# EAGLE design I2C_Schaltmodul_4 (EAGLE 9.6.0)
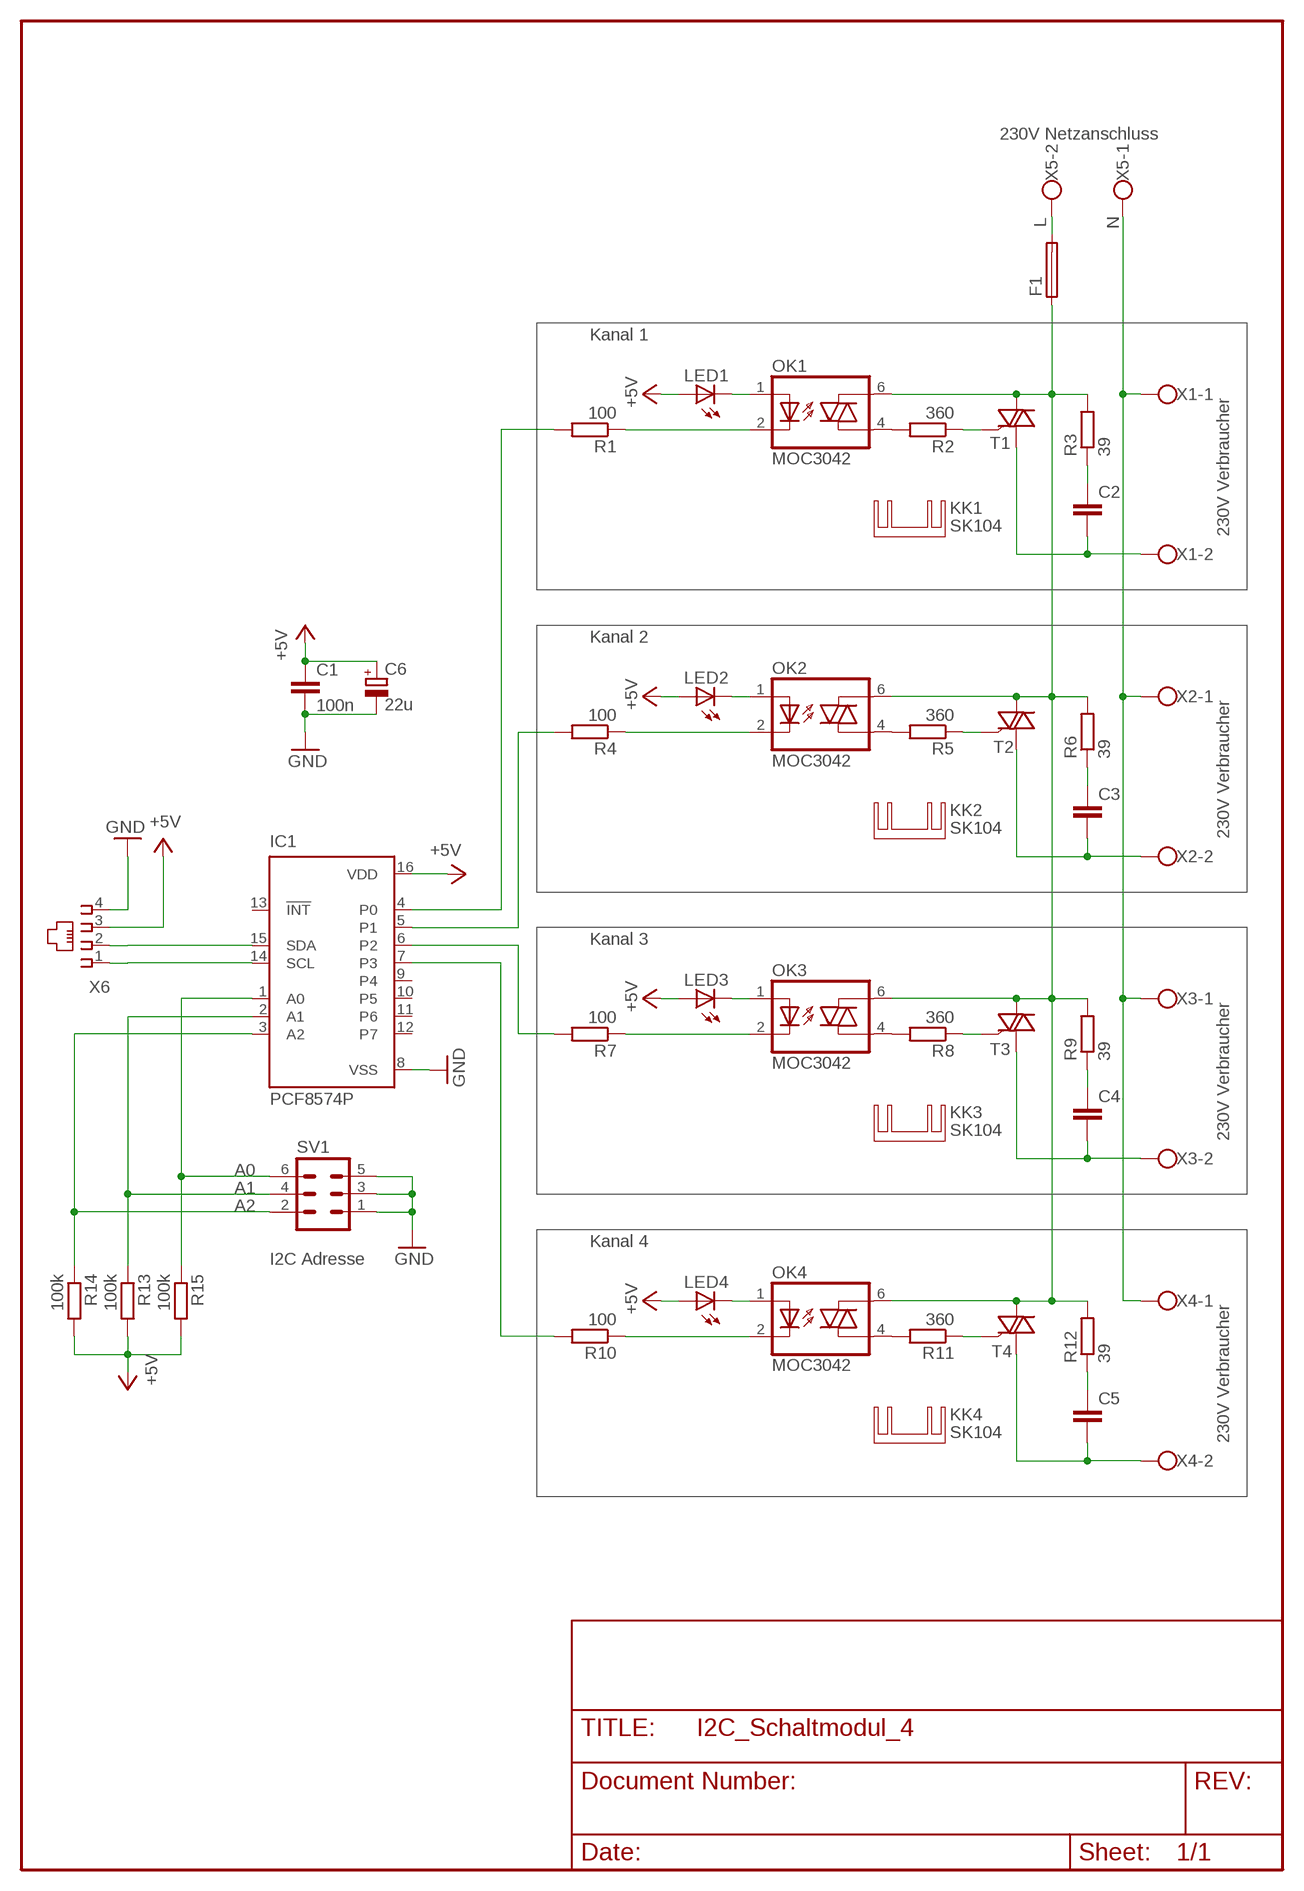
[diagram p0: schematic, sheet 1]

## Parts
C1  100n  C-EU075-032X103  [C075-032X103]
C2  C-EU102-043X133  [C102-043X133]
C3  C-EU102-043X133  [C102-043X133]
C4  C-EU102-043X133  [C102-043X133]
C5  C-EU102-043X133  [C102-043X133]
C6  22u  CPOL-EUE2.5-5  [E2,5-5]
F1  SH25  [SH25]
IC1  PCF8574P  [DIL16]
KK1  SK104  [SK104]
KK2  SK104  [SK104]
KK3  SK104  [SK104]
KK4  SK104  [SK104]
LED1  LED3MM  [LED3MM]
LED2  LED3MM  [LED3MM]
LED3  LED3MM  [LED3MM]
LED4  LED3MM  [LED3MM]
OK1  MOC3042  IL420  [DIL06]
OK2  MOC3042  IL420  [DIL06]
OK3  MOC3042  IL420  [DIL06]
OK4  MOC3042  IL420  [DIL06]
R1  100  R-EU_0207/10  [0207/10]
R2  360  R-EU_0207/10  [0207/10]
R3  39  R-EU_0411/15  [0411/15]
R4  100  R-EU_0207/10  [0207/10]
R5  360  R-EU_0207/10  [0207/10]
R6  39  R-EU_0411/15  [0411/15]
R7  100  R-EU_0207/10  [0207/10]
R8  360  R-EU_0207/10  [0207/10]
R9  39  R-EU_0411/15  [0411/15]
R10  100  R-EU_0207/10  [0207/10]
R11  360  R-EU_0207/10  [0207/10]
R12  39  R-EU_0411/15  [0411/15]
R13  100k  R-EU_0207/10  [0207/10]
R14  100k  R-EU_0207/10  [0207/10]
R15  100k  R-EU_0207/10  [0207/10]
SV1  MA03-2  [MA03-2]
T1  TIC225SBVH  [TO220BVH]
T2  TIC225SBVH  [TO220BVH]
T3  TIC225SBVH  [TO220BVH]
T4  TIC225SBVH  [TO220BVH]
X1  W237-102  [W237-102]
X2  W237-102  [W237-102]
X3  W237-102  [W237-102]
X4  W237-102  [W237-102]
X5  W237-102  [W237-102]
X6  215876-6  [215876-6]

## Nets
+5V: C1.1 C6.+ IC1.16(VDD) LED1.A LED2.A LED3.A LED4.A R13.2 R14.2 R15.2 X6.3
A0: IC1.1(A0) R15.1 SV1.6
A1: IC1.2(A1) R13.1 SV1.4
A2: IC1.3(A2) R14.1 SV1.2
GND: C1.2 C6.- IC1.8(VSS) SV1.1 SV1.3 SV1.5 X6.4
L: F1.2 X5.2
N: X1.1 X2.1 X3.1 X4.1 X5.1
N$1: IC1.4(P0) R1.2
N$2: LED1.K(C) OK1.1(A)
N$3: OK1.4(A1) R2.2
N$4: IC1.5(P1) R4.2
N$5: R2.1 T1.3(G)
N$6: C2.1 R3.1
N$7: OK1.2(C) R1.1
N$8: OK2.4(A1) R5.2
N$9: OK3.4(A1) R8.2
N$10: OK4.4(A1) R11.2
N$11: C3.2 T2.1(A1) X2.2
N$12: C3.1 R6.1
N$13: C2.2 T1.1(A1) X1.2
N$14: LED2.K(C) OK2.1(A)
N$15: OK2.2(C) R4.1
N$16: R5.1 T2.3(G)
N$17: C4.2 T3.1(A1) X3.2
N$18: C4.1 R9.1
N$19: IC1.6(P2) R7.2
N$20: LED3.K(C) OK3.1(A)
N$21: OK3.2(C) R7.1
N$22: R11.1 T4.3(G)
N$24: C5.2 T4.1(A1) X4.2
N$25: C5.1 R12.1
N$26: IC1.7(P3) R10.2
N$27: LED4.K(C) OK4.1(A)
N$28: OK4.2(C) R10.1
N$29: R8.1 T3.3(G)
N$100: F1.1 OK1.6(A2) OK2.6(A2) OK3.6(A2) OK4.6(A2) R3.2 R6.2 R9.2 R12.2 T1.2(A2) T2.2(A2) T3.2(A2) T4.2(A2)
SCL: IC1.14(SCL) X6.2
SDA: IC1.15(SDA) X6.1
Unconnected: IC1.9(P4) IC1.10(P5) IC1.11(P6) IC1.12(P7) IC1.13(!INT)

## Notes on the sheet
- 230V Netzanschluss
- Kanal 1
- 230V Verbraucher
- Kanal 2
- 230V Verbraucher
- Kanal 3
- 230V Verbraucher
- Kanal 4
- I2C Adresse
- 230V Verbraucher

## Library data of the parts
C1-C5 = rcl:C-EU: CAPACITOR, European symbol
C6 = rcl:CPOL-EU: POLARIZED CAPACITOR, European symbol
F1 = fuse:SH25: FUSE HOLDER
IC1 = micro-philips:PCF8574: I2C-Bus I/O DEVICE
KK1-KK4 = heatsink:SK104: HEATSINK
LED1-LED4 = led:LED: LED
OK1-OK4 = optocoupler:IL420: SIEMENS OPTO COUPLER
R1-R15 = rcl:R-EU_: RESISTOR, European symbol
SV1 = con-lstb:MA03-2: PIN HEADER
T1-T4 = selfmade:TIC225S: TRIAC
X1-X5 = con-wago-500:W237-102: WAGO SCREW CLAMP
X6 = con-amp:215876-6: AMP connector

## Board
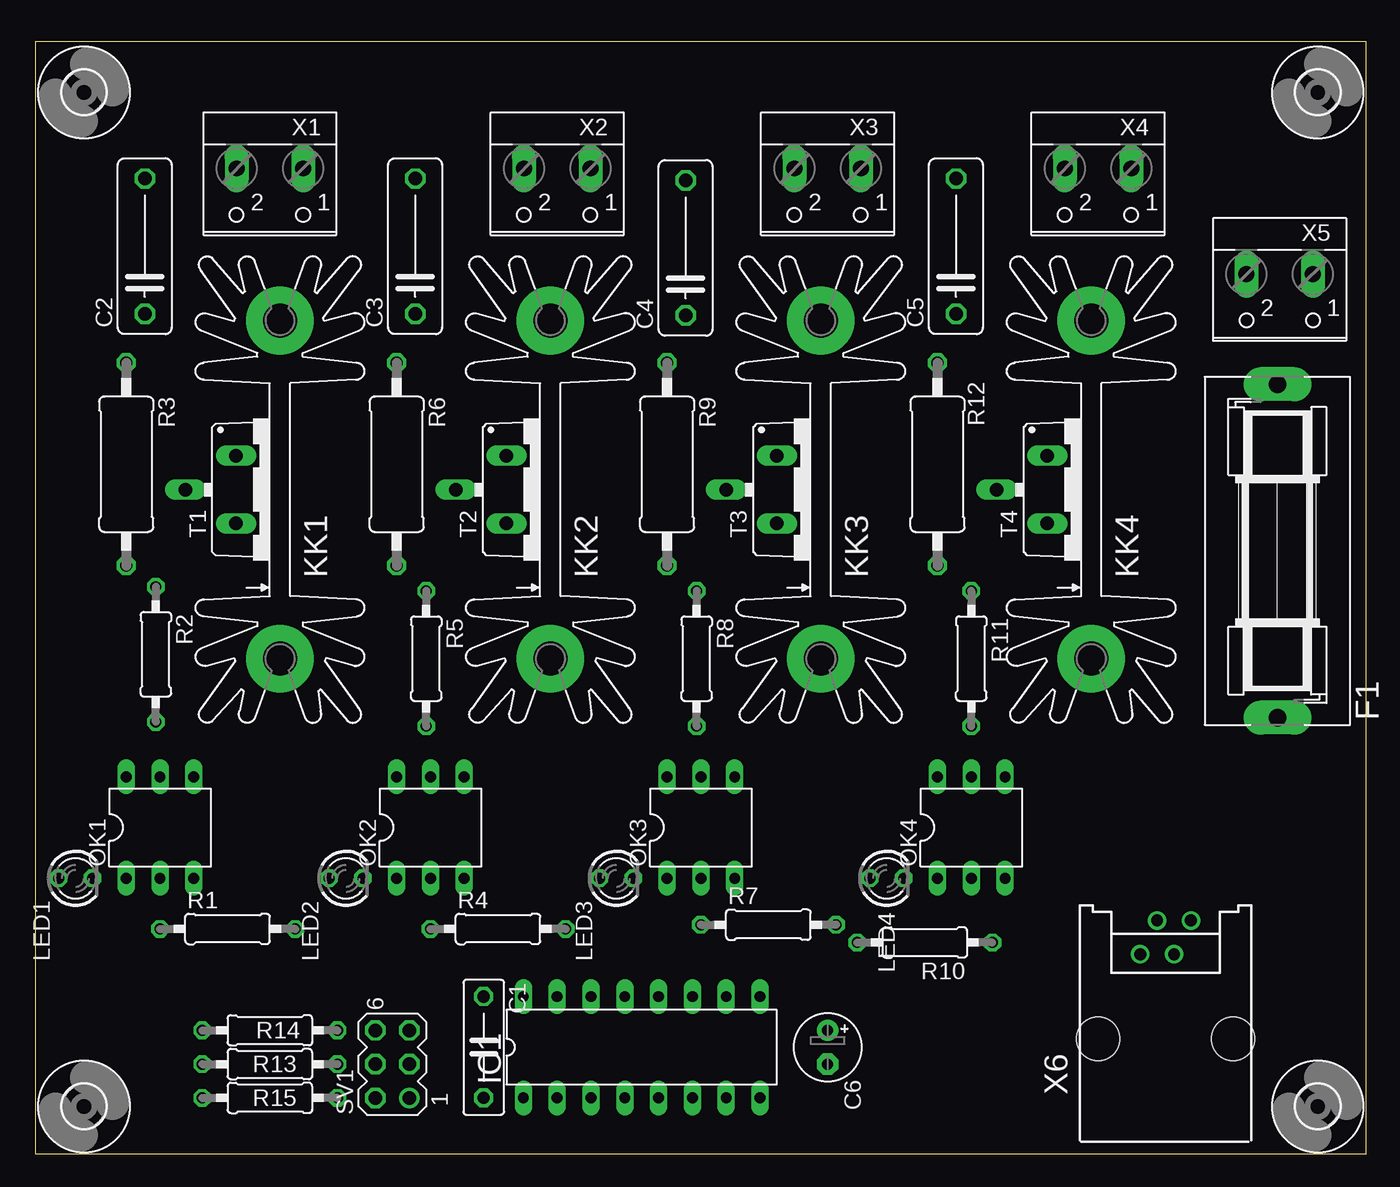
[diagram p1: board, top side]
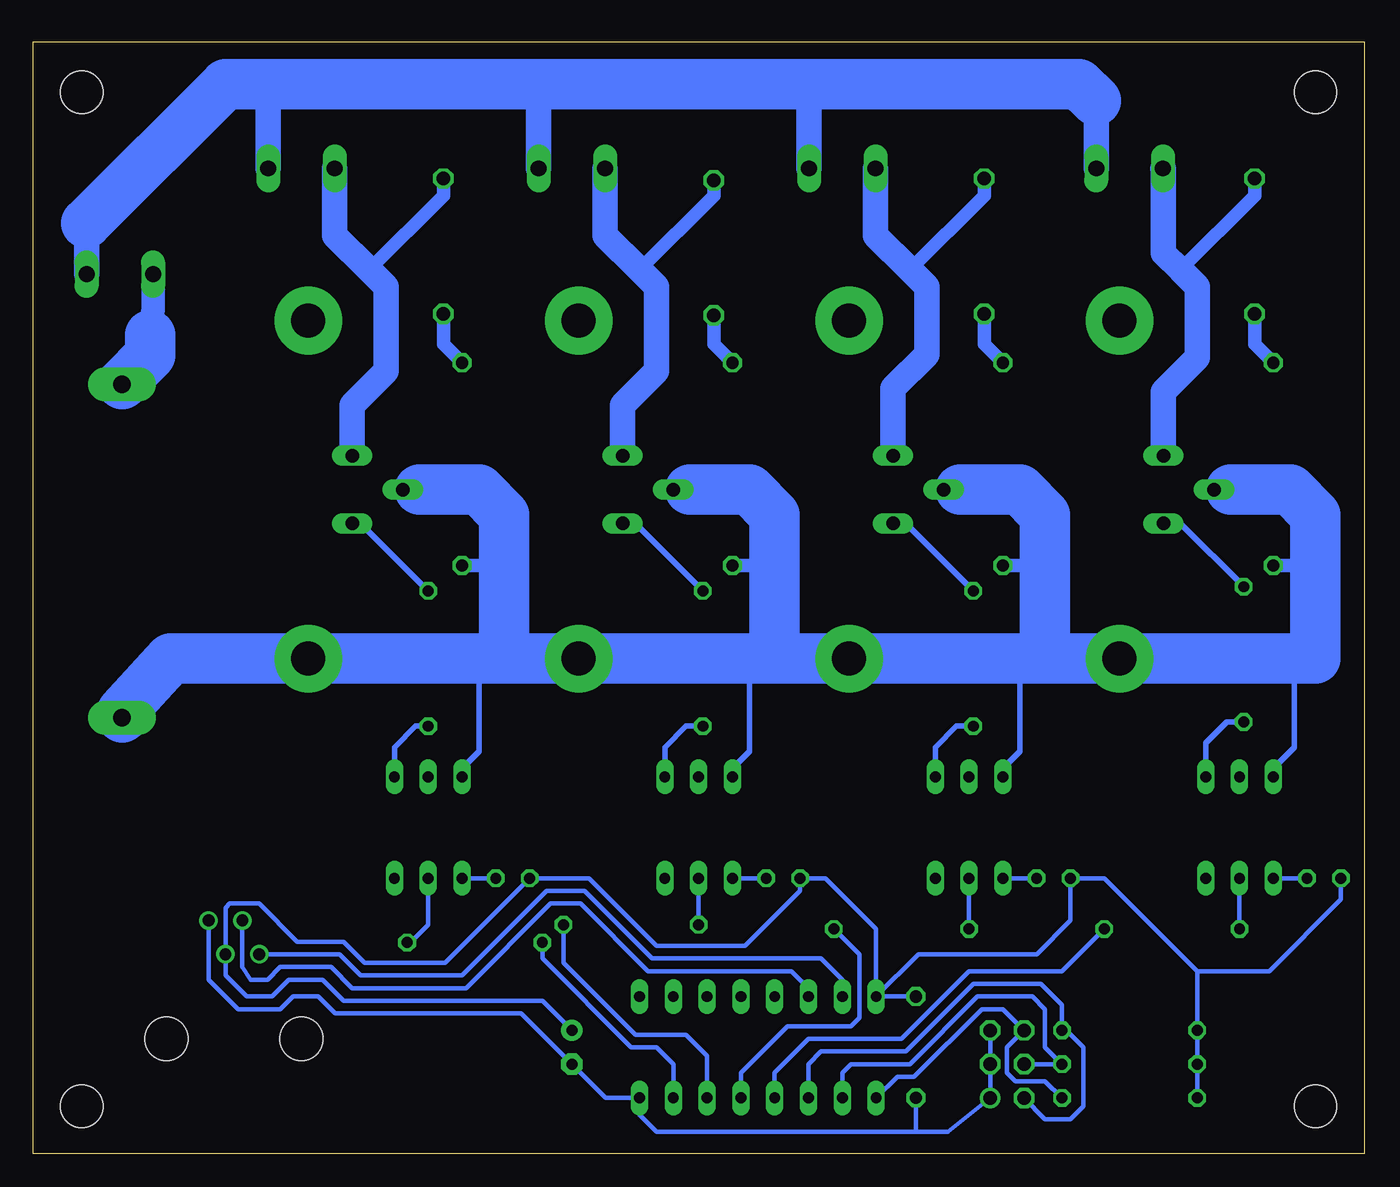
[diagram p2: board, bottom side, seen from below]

Size 100 x 83.56 mm. Coordinates in mm from the lower left corner, seen from the top.
Outline: 0,0 100,0 100,83.56 0,83.56 0,0
Copper layers (1*16): Top 0.035mm / dielectric 1.5mm / Bottom 0.035mm
Design rules "default": minimum track width 12mil, minimum drill 24mil, track to track 12mil, track to pad 12mil, pad to pad 12mil, via to via 12mil, smd to smd 8mil, copper to edge 40mil, drill to drill 8mil, minimum pad ring 10mil, minimum via ring 8mil, stop-mask expansion 4mil, vias tented up to drill 0mil, thermal gap 10mil

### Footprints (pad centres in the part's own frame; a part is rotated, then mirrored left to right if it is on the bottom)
C075-032X103 = drill 0.914 octagon: 1 -3.81,0; 2 3.81,0
C102-043X133 = drill 1.016 octagon: 1 -5.08,0; 2 5.08,0
E2,5-5 = drill 0.813 pad 1.6: + -1.27,0 | drill 0.813 pad 1.6 octagon: - 1.27,0
SH25 = drill 1.321 pad 2.54 long: 1 -12.522,0; 2 12.522,0
DIL16 = drill 0.813 long: 1 -8.89,-3.81; 2 -6.35,-3.81; 3 -3.81,-3.81; 4 -1.27,-3.81; 5 1.27,-3.81; 6 3.81,-3.81; 7 6.35,-3.81; 8 8.89,-3.81; 9 8.89,3.81; 10 6.35,3.81; 11 3.81,3.81; 12 1.27,3.81; 13 -1.27,3.81; 14 -3.81,3.81; 15 -6.35,3.81; 16 -8.89,3.81
SK104 = drill 2.54 pad 5.08: A2,5 -12.7,-0.762; B2,5 12.7,-0.762
LED3MM = drill 0.813 octagon: A -1.27,0; K 1.27,0
DIL06 = drill 0.813 long: 1 -2.54,-3.81; 2 0,-3.81; 3 2.54,-3.81; 4 2.54,3.81; 5 0,3.81; 6 -2.54,3.81
0207/10 = drill 0.813 octagon: 1 -5.08,0; 2 5.08,0
0411/15 = drill 0.914 octagon: 1 -7.62,0; 2 7.62,0
MA03-2 = drill 1.016: 1 -2.54,-1.27 | drill 1.016 octagon: 2 -2.54,1.27; 3 0,-1.27; 4 0,1.27; 5 2.54,-1.27; 6 2.54,1.27
TO220BVH = drill 1.016 long: 1 -2.54,-2.54; 2 0,-6.35; 3 2.54,-2.54
3,2 = hole 3.2: 0,0
W237-102 = drill 1.194 long: 1 -2.5,-1.27; 2 2.5,-1.27
215876-6 = drill 0.889: 1 -1.905,6.35; 2 -0.635,8.89; 3 0.635,6.35; 4 1.905,8.89 | hole 3.251: -5.08,0; 5.08,0

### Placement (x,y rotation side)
C1  33.68,8 270 top
C2  8.22,68.19 90 top
C3  28.54,68.19 90 top
C4  48.86,68.07 90 top
C5  69.18,68.19 90 top
C6  59.52,8 270 top
F1  93.33,45.3 90 top
IC1  45.55,8 0 top
KK1  17.61,49.91 90 top
KK2  37.94,49.91 90 top
KK3  58.25,49.91 90 top
KK4  78.58,49.91 90 top
LED1  3.01,20.7 0 top
LED2  23.33,20.7 0 top
LED3  43.65,20.7 0 top
LED4  63.97,20.7 0 top
OK1  9.36,24.51 0 top
OK2  29.68,24.51 0 top
OK3  50,24.51 0 top
OK4  70.32,24.51 0 top
R1  14.44,16.89 0 top
R2  9.04,37.52 270 top
R3  6.82,51.81 270 top
R4  34.76,16.89 0 top
R5  29.36,37.21 270 top
R6  27.14,51.81 270 top
R7  55.08,17.2 0 top
R8  49.68,37.21 270 top
R9  47.46,51.81 270 top
R10  66.83,15.87 180 top
R11  70.32,37.21 270 top
R12  67.78,51.81 270 top
R13  17.61,6.73 180 top
R14  17.61,9.27 180 top
R15  17.61,4.19 180 top
SV1  26.82,6.73 90 top
T1  17.61,49.91 270 top
T2  37.94,49.91 270 top
T3  58.25,49.91 270 top
T4  78.58,49.91 270 top
U$1  [3,2]  3.64,3.55 0 top
U$2  [3,2]  96.36,3.55 0 top
U$3  [3,2]  96.36,79.75 0 top
U$4  [3,2]  3.64,79.75 0 top
X1  17.61,72.77 180 top
X2  39.2,72.77 180 top
X3  59.52,72.77 180 top
X4  79.84,72.77 180 top
X5  93.5,64.83 180 top
X6  84.92,8.63 0 top

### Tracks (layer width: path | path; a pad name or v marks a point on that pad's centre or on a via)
+5V
  Bottom 0.356: R13.2 R15.2 R13.2 | 12.54,13.71 R14.2 R13.2 | IC1.16 33.49,14.98 24.6,14.98 22.06,17.52 LED2.A 19.52,20.7 12.54,13.71 | IC1.16 36.66,16.89 40.48,20.7 LED3.A 42.38,19.74 46.51,15.62 53.17,15.62 58.25,20.7 LED4.A 69.05,14.35 75.08,14.35 76.67,15.93 80.16,15.93 83.02,18.79 85.24,18.79 85.56,18.47 X6.3 85.56,13.39 83.97,11.81 82.07,11.81 80.8,13.08 78.26,13.08 76.67,11.49 61.75,11.49 C6.+ | LED1.A 1.74,19.11 7.14,13.71 12.54,13.71 | IC1.16 C1.1
A0
  Bottom 0.356: IC1.1 35.08,5.77 33.81,5.77 28.73,10.85 27.14,10.85 SV1.6 | SV1.6 25.55,8.95 | R15.1 23.96,5.46 26.19,5.46 26.82,6.09 26.82,8 SV1.6
A1
  Bottom 0.356: IC1.2 39.2,6.09 38.57,6.73 34.12,6.73 29.04,11.81 24.92,11.81 23.96,10.85 23.96,8 R13.1 SV1.4
A2
  Bottom 0.356: IC1.3 41.74,6.73 40.79,7.68 34.44,7.68 29.36,12.76 24.28,12.76 22.7,11.17 R14.1 22.38,9.27 21.11,8 21.11,3.55 22.06,2.6 23.96,2.6 SV1.2
GND
  Bottom 0.356: 33.81,1.65 31.27,1.65 SV1.1 SV1.3 | 33.81,1.65 53.17,1.65 54.45,2.92 IC1.8 56.98,4.19 C6.- 63.34,10.54 77.3,10.54 78.58,11.81 80.48,11.81 81.43,10.85 84.61,10.85 86.83,13.08 X6.4 | SV1.3 SV1.5 SV1.3 | C1.2 33.68,1.77 33.81,1.65
L
  Bottom 1.778: X5.2 91,63.52 91.21,61.53
  Bottom 3.81: 91.21,61.53 91.21,60 93.33,57.89 F1.2
N
  Bottom 1.93: X5.1 96,69.87 96.04,69.91 | 20.15,79.12 20.15,78.8 20.11,78.76 X1.1 | X2.1 41.7,80.03 42.06,80.39 | X3.1 62.02,79.71 62.06,79.75 62.06,80.39 61.75,80.7 61.75,80.39 | 82.7,80.39 82.7,80.07 82.34,79.71 X4.1
  Bottom 3.81: 96.04,69.91 85.56,80.39 82.7,80.39 61.75,80.39 42.06,80.39 21.42,80.39 20.15,79.12
N$1
  Bottom 0.356: R1.2 22.7,13.71 29.68,13.71 34.76,8.63 41.74,8.63 44.28,6.09 IC1.4
N$2
  Bottom 0.356: LED1.K OK1.1
N$3
  Bottom 0.406: OK1.4 11.9,30.86 10.31,32.44 R2.2
N$4
  Bottom 0.356: R4.2 37.94,14.98 37.94,10.22 38.57,9.58 43.33,9.58 46.82,6.09 IC1.5
N$5
  Bottom 0.406: T1.3 13.81,47.37 R2.1
N$6
  Bottom 1.016: C2.1 8.22,60.83 R3.1
N$7
  Bottom 0.356: R1.1 OK1.2
N$8
  Bottom 0.406: OK2.4 32.22,30.54 30.63,32.13 R5.2
N$9
  Bottom 0.406: OK3.4 52.54,30.54 50.95,32.13 R8.2
N$10
  Bottom 0.406: OK4.4 72.86,30.54 71.27,32.13 R11.2
N$11
  Bottom 1.016: 34.12,66.42 28.54,72 C3.2 | T2.1 35.39,52.95
  Bottom 1.93: 35.39,52.95 35.39,57.53 32.85,60.07 32.85,65.15 34.12,66.42 36.7,69 X2.2
N$12
  Bottom 1.016: C3.1 28.54,60.83 R6.1
N$13
  Bottom 1.016: C2.2 8.22,72 13.81,66.42 | T1.1 15.08,52.95
  Bottom 1.93: 15.08,52.95 15.08,57.27 12.54,59.81 12.54,65.15 13.81,66.42 15.08,67.69 15.08,74.04 X1.2
N$14
  Bottom 0.356: LED2.K OK2.1
N$15
  Bottom 0.356: R4.1 OK2.2
N$16
  Bottom 0.406: T2.3 34.44,47.37 R5.1
N$17
  Bottom 1.016: 54.45,66.42 48.86,72 C4.2 | T3.1 55.71,52.95
  Bottom 1.93: 55.71,52.95 55.71,56.26 53.17,58.8 53.17,65.15 54.45,66.42 57.02,69 X3.2
N$18
  Bottom 1.016: C4.1 48.86,60.83 R9.1
N$19
  Bottom 0.356: R7.2 60.16,14.35 54.76,8.95 50.95,8.95 49.37,7.36 IC1.6
N$20
  Bottom 0.356: LED3.K OK3.1
N$21
  Bottom 0.356: R7.1 OK3.2
N$22
  Bottom 0.406: T4.3 75.4,47.37 R11.1
N$24
  Bottom 1.016: 74.77,66.42 69.18,72 C5.2 | T4.1 76.03,52.95
  Bottom 1.93: 76.03,52.95 76.03,56.26 73.5,58.8 73.5,65.15 74.77,66.42 77.34,69 X4.2
N$25
  Bottom 1.016: C5.1 69.18,60.83 R12.1
N$26
  Bottom 0.356: IC1.7 51.91,6.73 53.17,8 55.08,8 61.75,14.66 R10.2
N$27
  Bottom 0.356: LED4.K OK4.1
N$28
  Bottom 0.356: R10.1 71.65,15.87 70.32,17.2 OK4.2
N$29
  Bottom 0.406: T3.3 54.76,47.37 R8.1
N$100
  Bottom 0.406: OK4.6 67.78,28.95 66.51,30.22 66.51,37.21 | OK3.6 47.46,28.95 46.19,30.22 46.19,37.21 | OK2.6 27.14,28.95 25.87,30.22 25.87,37.21 | OK1.6 6.82,28.95 5.23,30.54 5.23,37.21
  Bottom 1.016: 3.64,44.19 R3.2 | 23.96,44.19 R6.2 | 44.28,44.19 R9.2 | 64.61,44.19 R12.2 | 10,49.91 T1.2 | 30.31,49.91 T2.2 25.87,49.91 23.33,46.73 23.33,37.21 | 50.63,49.91 T3.2 | 70.95,49.91 T4.2 72.86,49.91
  Bottom 3.81: F1.1 93.33,33.25 89.69,37.21 66.51,37.21 64.61,37.21 | 44.28,37.21 46.19,37.21 64.61,37.21 | 23.96,37.84 23.96,44.19 23.96,48 25.87,49.91 30.31,49.91 | 44.28,37.21 44.28,44.19 44.28,48 46.19,49.91 50.63,49.91 | 64.61,37.21 64.61,44.19 64.61,48 66.51,49.91 70.95,49.91 | 44.28,37.21 25.87,37.21 23.33,37.21 5.23,37.21 3.64,37.21 3.64,44.19 3.64,48 5.55,49.91 10,49.91
SCL
  Bottom 0.356: IC1.14 41.74,12.44 43.02,13.71 53.81,13.71 58.89,18.79 61.11,18.79 67.46,12.44 76.03,12.44 77.62,14.03 81.43,14.03 82.39,13.08 83.66,13.08 84.29,14.03 X6.2
SDA
  Bottom 0.356: IC1.15 39.2,13.08 40.79,14.66 53.49,14.66 58.57,19.74 61.43,19.74 67.78,13.39 75.4,13.39 76.99,14.98 X6.1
